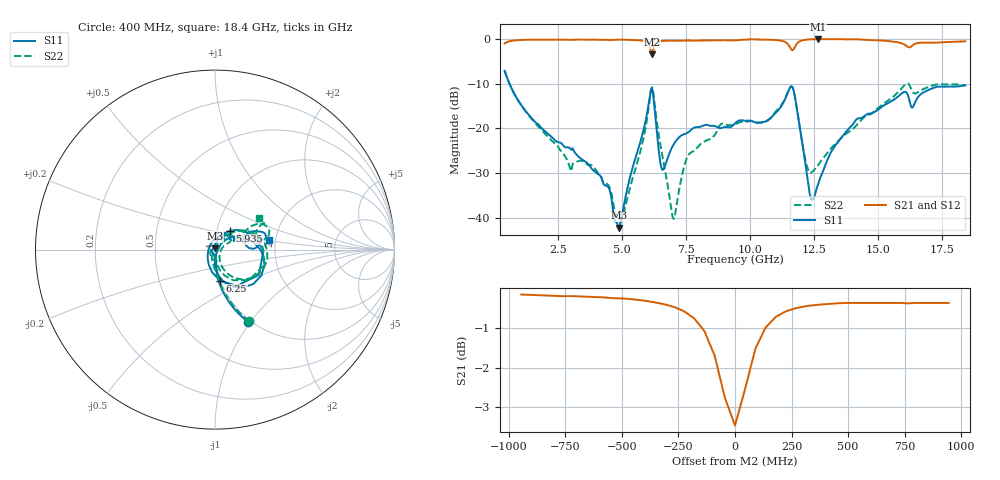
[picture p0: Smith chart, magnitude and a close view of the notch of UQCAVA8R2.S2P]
!  Part Number  UQCAVA8R2
!  Description: RF capacitor  Mounting Orientation: Horizontal
!  Application:
# GHZ S DB R 50
! Freq  |S11|  S11 Ph  |S21|  S21 Ph  |S12|  S12 Ph  |S22|  S22 Ph
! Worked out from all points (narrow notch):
!   401 points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, 400 MHz to 18.4 GHz, reference 50 ohm
!   highest |S21| = 0.00 dB at 12.64 GHz (marker M1); lowest = -3.5 dB at 6.16 GHz (marker M2)
!   notch at M2: 3.2 dB deep, 160 MHz wide at half that depth
!   lowest |S11| = -42.2 dB at 4.855 GHz (marker M3), VSWR 1.02, Z = 50 + j0.77 ohm
!   |S11| at or under -10 dB: 589.9 MHz to end of sweep
!   |S22| runs from -41.1 to -7.1 dB; largest |S21 - S12| = 0.0023
!   S11 on the Smith chart (normalised r, x): 400 MHz: 0.97, -0.97; 5.935 GHz: 1.15, +0.24; 6.25 GHz: 0.99, -0.35; 18.4 GHz: 1.83, +0.22
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0.4  -7.09 -65.5  -0.98 24.6  -0.99 24.6  -7.09 -64.4
1.39  -17.29 -85.5  -0.14 2.1  -0.14 2.1  -17.45 -86.8
2.92  -24.32 -86.1  -0.18 -8.7  -0.18 -8.6  -28.26 -115.5
3.415  -26.95 -91.7  -0.11 -11.2  -0.11 -11.2  -27.28 -114.4
4.45  -33.15 -131.4  -0.20 -16.8  -0.20 -16.7  -32.69 -173.1
4.855  -42.25 92.9  -0.12 -18.6  -0.12 -18.5  -40.79 122.1
5.935  -17.57 51.7  -0.59 -29.2  -0.59 -29.1  -18.91 50.4
6.16  -11.00 -29.6  -3.45 -22.2  -3.45 -22.2  -10.79 -16.9
6.25  -15.17 -81.1  -1.53 -13.4  -1.53 -13.3  -13.99 -59.0
6.43  -25.45 -139.5  -0.51 -19.1  -0.50 -19.1  -21.77 -82.2
6.61  -29.16 147.2  -0.39 -21.8  -0.39 -21.8  -27.68 -82.1
7.015  -23.48 83.4  -0.38 -24.7  -0.38 -24.7  -40.30 -5.4
7.6  -20.77 58.9  -0.32 -27.8  -0.31 -27.7  -25.81 45.7
9.4  -18.89 39.3  -0.30 -35.2  -0.30 -35.2  -19.08 44.2
10.705  -18.16 27.4  -0.14 -43.1  -0.14 -43.1  -18.04 44.6
11.605  -10.58 -29.1  -2.38 -47.9  -2.37 -47.9  -10.53 -11.6
12.19  -29.53 -82.5  -0.12 -42.9  -0.11 -43.0  -28.07 -49.3
12.415  -35.96 -24.9  -0.04 -45.2  -0.03 -45.2  -29.72 -10.8
12.64  -32.60 22.1  0.00 -47.0  -0.01 -47.0  -28.30 8.8
14.08  -18.49 37.8  -0.05 -55.2  -0.04 -55.2  -19.71 29.9
15.43  -14.17 24.7  -0.47 -63.3  -0.46 -63.3  -13.59 32.2
18.4  -10.36 10.2  -0.50 -72.5  -0.50 -72.5  -10.39 35.4
